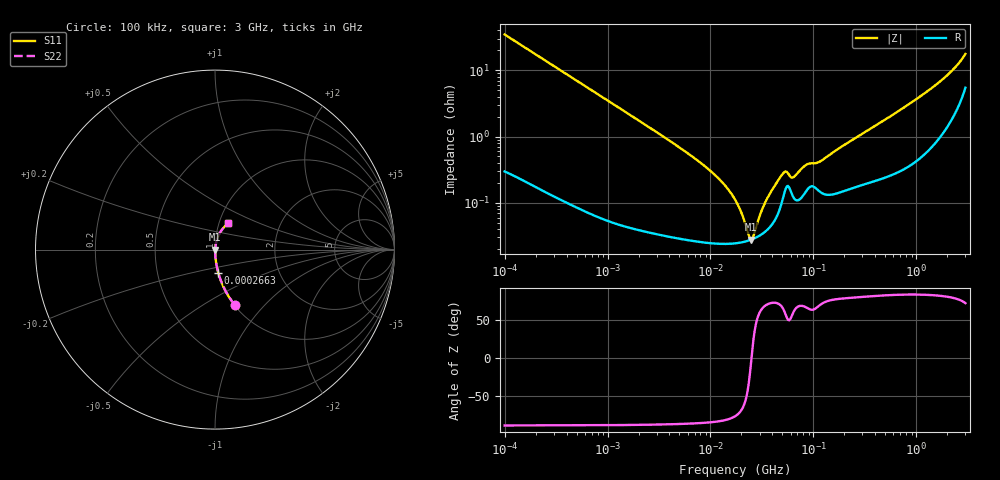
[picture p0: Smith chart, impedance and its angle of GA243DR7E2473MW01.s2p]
!Murata Part Number: GA243DR7E2473MW01
!These Parameters are Measured in Series Mode Connection
!Data Generated on Jun 19, 2026
!  o--ll--o
!Port1  Port2
!  o------o
!Operation Temp=25[degC], DC Bias Voltage=0[V]
!Freq. Start=100[kHz] Stop=3[GHz] 401[Steps]
# Hz S RI R 50
!Freq.(Hz) S11(Real) S11(Imag) S21(Real) S21(Imag) S12(Real) S12(Imag) S22(Real) S22(Imag)
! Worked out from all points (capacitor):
!   401 points, 100 kHz to 3 GHz, reference 50 ohm
!   read as one part in series: C = 45.9 nF near 105.3 kHz
!   lowest |Z| = 27.9 mohm at 24.85 MHz (marker M1)
!   series resonance near 25.06 MHz, so ESL is about 880 pH
!   S11 on the Smith chart (normalised r, x): 100 kHz: 1.01, -0.69; 266.3 kHz: 1.00, -0.26; 3 GHz: 1.11, +0.34
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100000  0.1092 -0.3077  0.8908 0.3077  0.8908 0.3077  0.1092 -0.3077
266273  0.0181 -0.1283  0.9819 0.1283  0.9819 0.1283  0.0181 -0.1283
562235  0.00463 -0.0619  0.9954 0.0619  0.9954 0.0619  0.00463 -0.0619
3161081  0.000452 -0.011  0.9995 0.011  0.9995 0.011  0.000452 -0.011
1.008119e7  0.000255 -0.00299  0.9997 0.00299  0.9997 0.00299  0.000255 -0.00299
1.409348e7  0.000243 -0.00175  0.9998 0.00175  0.9998 0.00175  0.000243 -0.00175
1.77727e7  0.000246 -0.00102  0.9998 0.00102  0.9998 0.00102  0.000246 -0.00102
2.021703e7  0.000254 -0.000631  0.9997 0.000631  0.9997 0.000631  0.000254 -0.000631
2.359795e7  0.00027 -0.000177  0.9997 0.000177  0.9997 0.000177  0.00027 -0.000177
2.484619e7  0.000278 -2.55e-05  0.9997 2.55e-05  0.9997 2.55e-05  0.000278 -2.55e-05
2.616047e7  0.000287 0.000127  0.9997 -0.000127  0.9997 -0.000127  0.000287 0.000127
3.053531e7  0.000326 0.000596  0.9997 -0.000596  0.9997 -0.000596  0.000326 0.000596
3.473492e7  0.000378 0.00101  0.9996 -0.00101  0.9996 -0.00101  0.000378 0.00101
4.982709e7  0.00107 0.00246  0.9989 -0.00246  0.9989 -0.00246  0.00107 0.00246
5.383243e7  0.00164 0.00248  0.9984 -0.00248  0.9984 -0.00248  0.00164 0.00248
6.447533e7  0.00119 0.00214  0.9988 -0.00214  0.9988 -0.00214  0.00119 0.00214
8.342988e7  0.00144 0.00336  0.9986 -0.00336  0.9986 -0.00336  0.00144 0.00336
9.738194e7  0.00179 0.00351  0.9982 -0.00351  0.9982 -0.00351  0.00179 0.00351
1.196798e8  0.00143 0.00408  0.9986 -0.00408  0.9986 -0.00408  0.00143 0.00408
5.475153e8  0.00291 0.0194  0.9971 -0.0194  0.9971 -0.0194  0.00291 0.0194
1.616196e9  0.0126 0.0615  0.9874 -0.0615  0.9874 -0.0615  0.0126 0.0615
3e9  0.075 0.147  0.925 -0.147  0.925 -0.147  0.075 0.147
